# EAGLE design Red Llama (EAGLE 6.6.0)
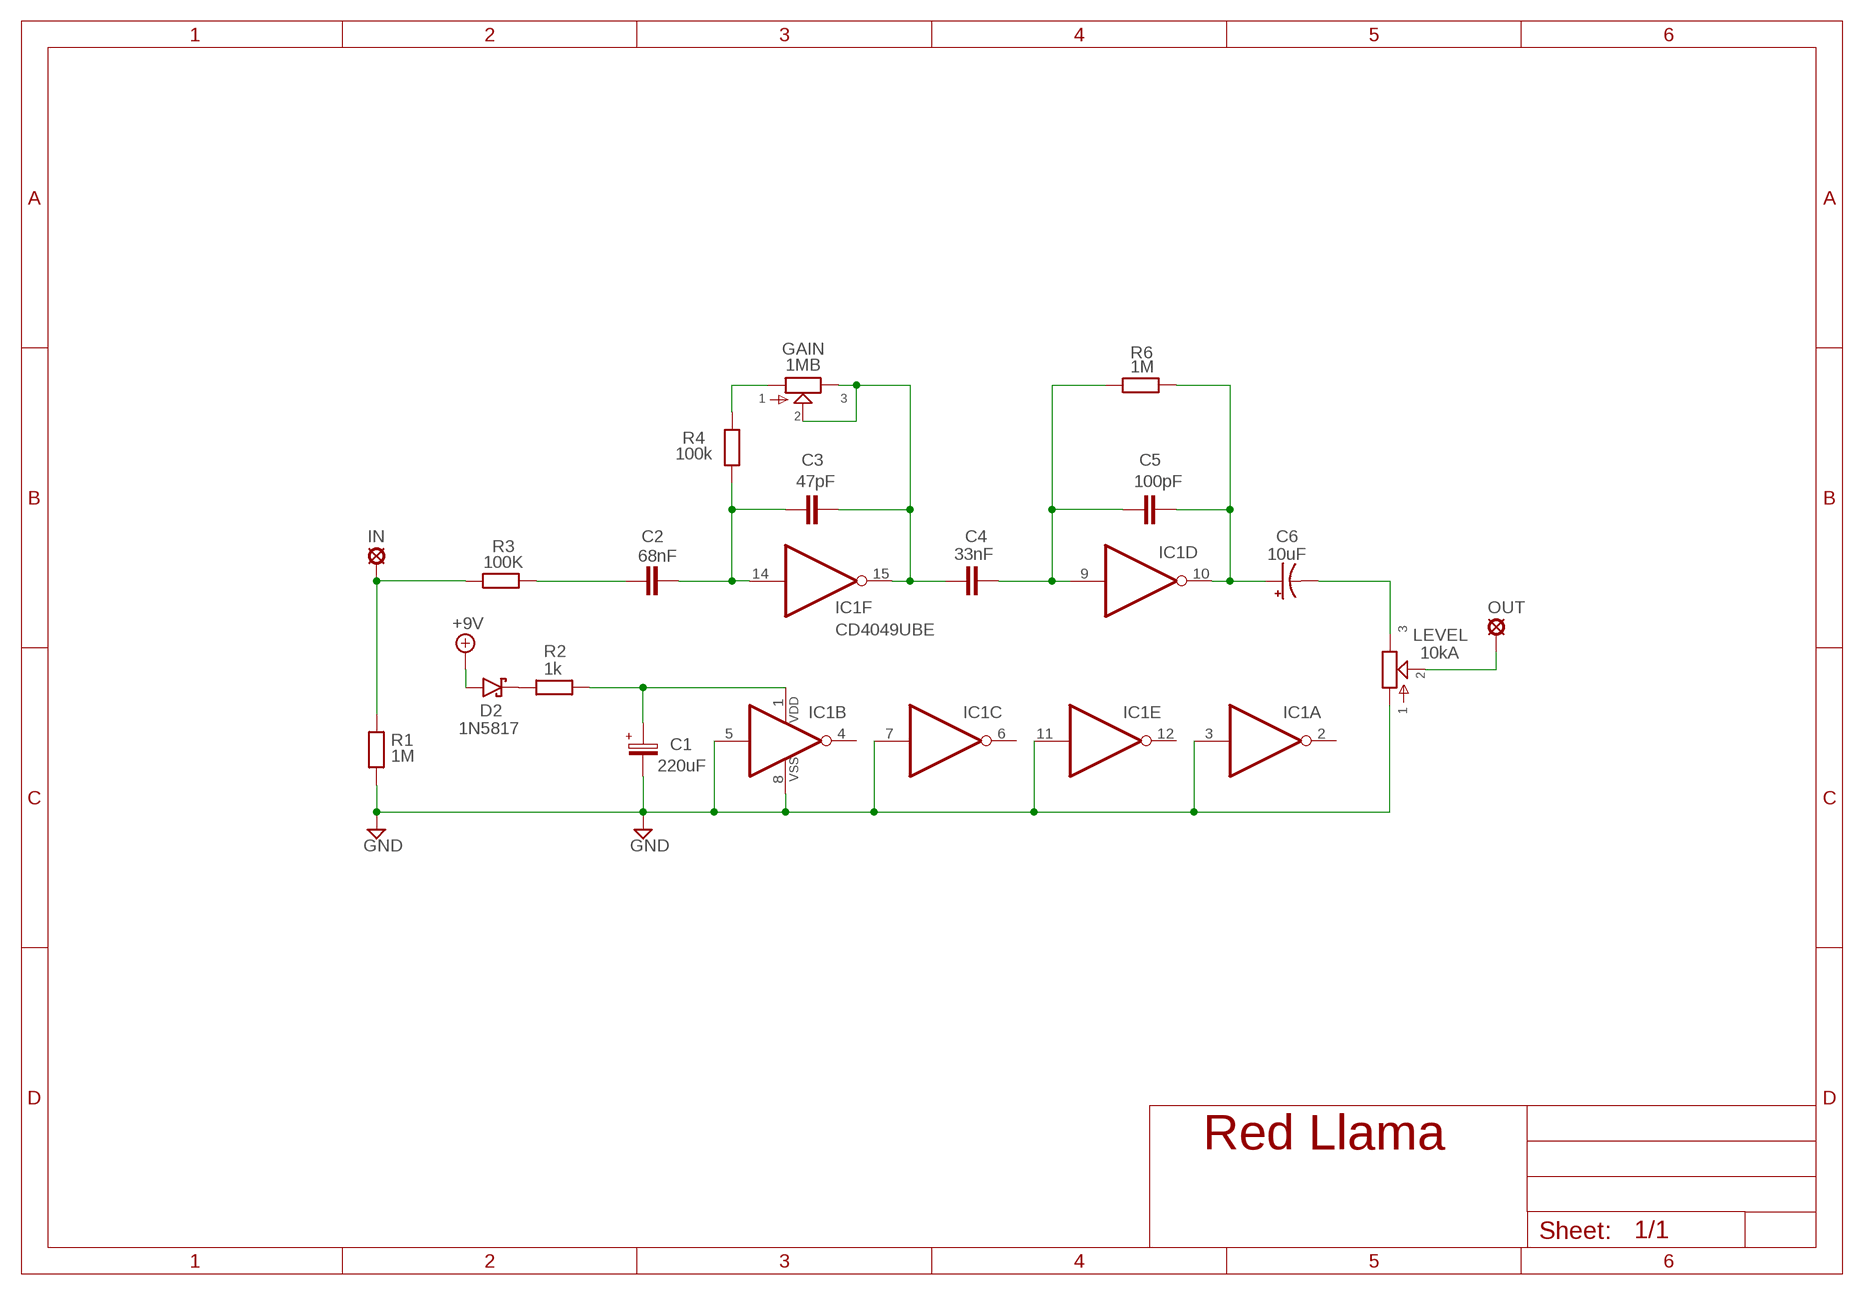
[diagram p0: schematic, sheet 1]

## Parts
+9V  +9V  +9V(T)1  [ROUND]
C1  220uF  063-EU  [063_025]
C2  68nF  10NF-47NF"  [4,5MM]
C3  47pF  050X030_0251  [050X030_025]
C4  33nF  10NF-47NF"  [4,5MM]
C5  100pF  050X030_0251  [050X030_025]
C6  10uF  044A2  [044A_2]
D2  1N5817  [DO41-3]
GAIN  1MB  POT-EU16MM  [16MM]
GND  GND  GND(T)1  [ROUND]
GND2  GND  GND(T)1  [ROUND]
IC1  CD4049UBE  [DIL16]
IN  MCS10B  [MCS10B]
LEVEL  10kA  POT-EU16MM  [16MM]
OUT  MCS10B  [MCS10B]
R1  1M  6MM-EU3  [R0207/3]
R2  1k  6MM-EU3  [R0207/3]
R3  100K  6MM-EU3  [R0207/3]
R4  100k  6MM-EU3  [R0207/3]
R6  1M  6MM-EU3  [R0207/3]

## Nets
+9V: +9V.1(+9V) D2.A
GND: C1.- GND2.1(GND) GND.1(GND) IC1.3(A:I) IC1.5(B:I) IC1.7(C:I) IC1.8(P:VSS) IC1.11(E:I) LEVEL.1 R1.1
N$1: LEVEL.2 OUT.MP
N$2: C4.2 C5.1 IC1.9(D:I) R6.1
N$3: IN.MP R1.2 R3.1
N$7: D2.C R2.1
N$8: GAIN.1 R4.2
N$9: C1.+ IC1.1(P:VDD) R2.2
N$18: C5.2 C6.1(+) IC1.10(D:O) R6.2
N$19: C3.2 C4.1 GAIN.2 GAIN.3 IC1.15(F:O)
N$20: C6.2(-) LEVEL.3
N$21: C2.2 C3.1 IC1.14(F:I) R4.1
N$24: C2.1 R3.2
Unconnected: IC1.2(A:O) IC1.4(B:O) IC1.6(C:O) IC1.12(E:O)

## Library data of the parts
+9V = gm-supply:+9V(T): +9V Voltage Supply
C1 = Elektrolyytit:063-EU
C2 C4 = Mylar Kondensaattorit:10NF-47NF: 10nF-47nF
C3 C5 = Keraamiset kondensaattorit:050X030_025: 47 - 120pF
C6 = gm-caps-tant:044A: .1 - 1.5µF
D2 = Diodit:1N5817
GAIN LEVEL = gm-pots:POT-EU
GND GND2 = gm-supply:GND(T): Ground
IC1 = Operaatiovahvistimet:CD4049UBE: Hex Inverting Buffer Used, for example, in the Red Llama, Three Legged Dog, and Hot Harmonics.
IN OUT = Padit:MCS10B: SOLDER PAD
R1-R4 R6 = Vastukset:6MM-EU: 6mm Resistors (European schematic symbol)

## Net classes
0 default: width 0.406 mm

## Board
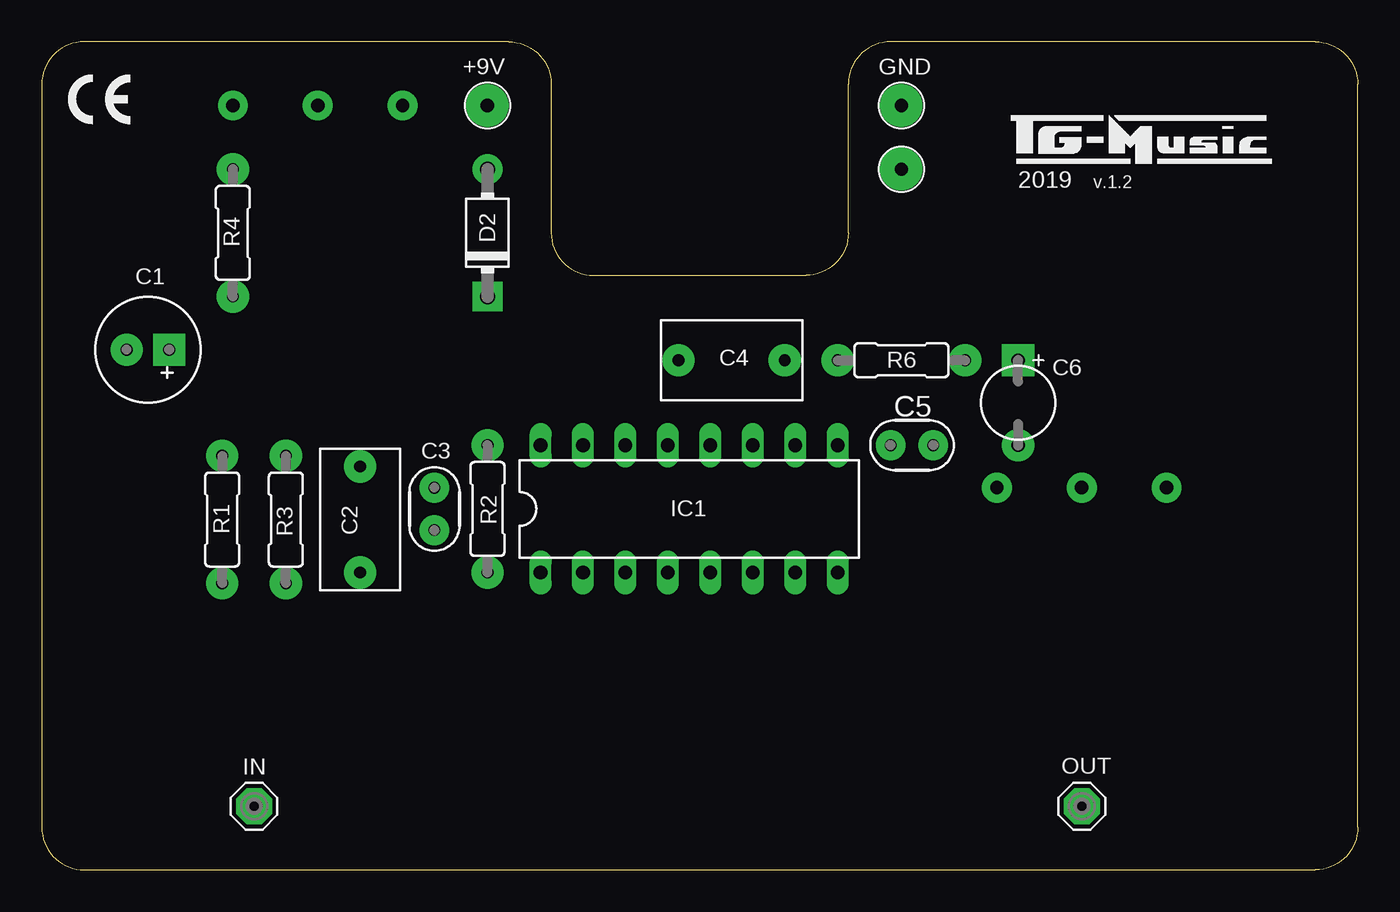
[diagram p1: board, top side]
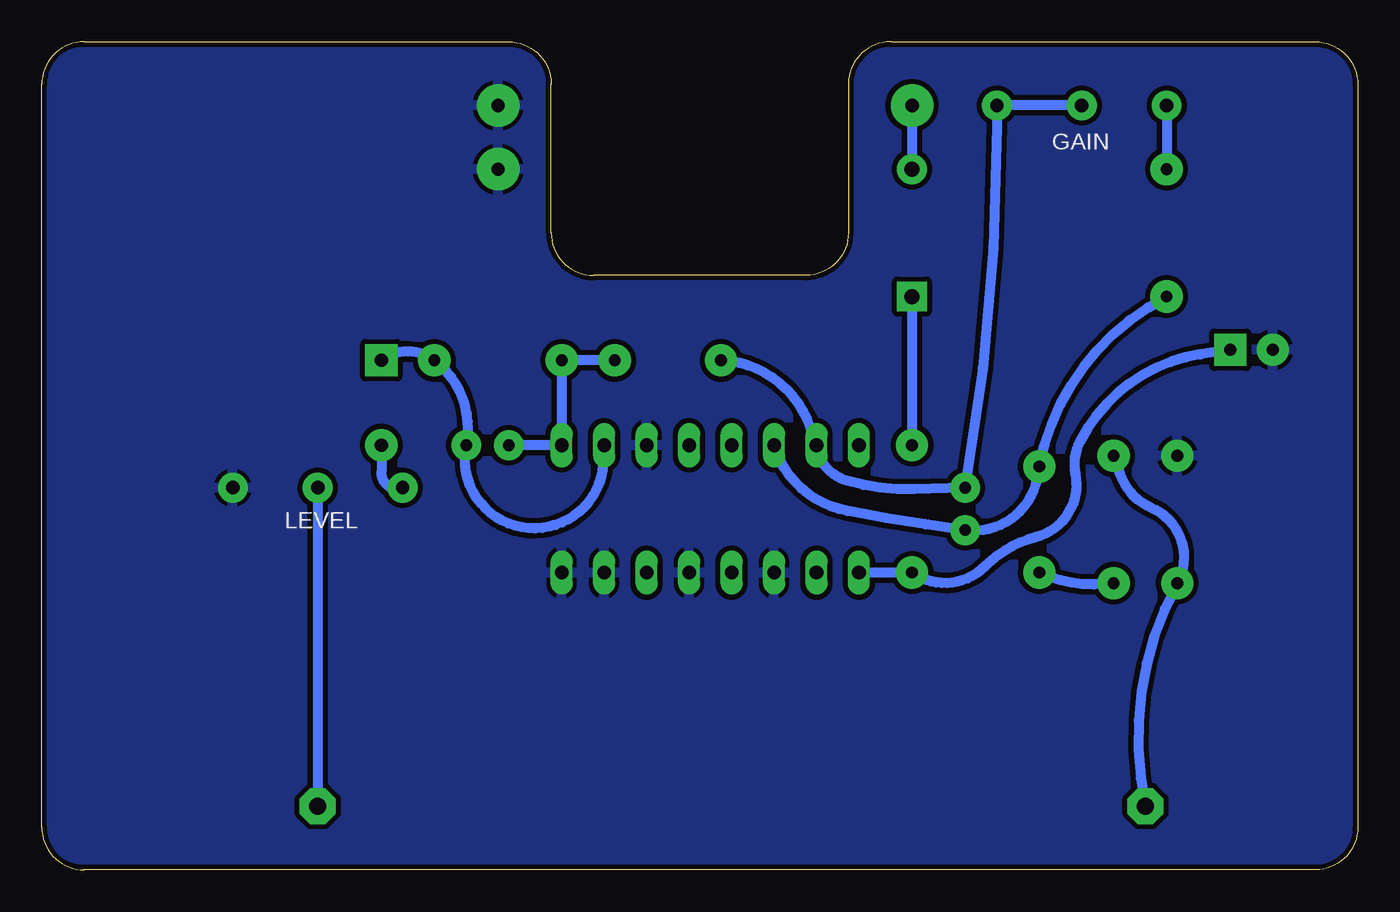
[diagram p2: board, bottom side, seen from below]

Size 78.74 x 49.53 mm. Coordinates in mm from the lower left corner, seen from the top.
Outline: 78.74,2.54 78.74,46.99 arc90 76.2,49.53 50.8,49.53 arc90 48.26,46.99 48.26,38.1 arc-90 45.72,35.56 33.02,35.56 arc-90 30.48,38.1 30.48,46.99 arc90 27.94,49.53 2.54,49.53 arc90 0,46.99 0,2.54 arc90 2.54,0 76.2,0 arc90 78.74,2.54
Copper layers (1*16): Top 0.035mm / dielectric 1.5mm / Bottom 0.035mm
Design rules "ITEADstudio": minimum track width 10mil, minimum drill 12mil, track to track 12mil, track to pad 12mil, pad to pad 12mil, via to via 12mil, smd to smd 0mil, copper to edge 12mil, drill to drill 12mil, minimum pad ring 10mil, minimum via ring 6mil, stop-mask expansion 4mil, vias tented up to drill 100mil, thermal gap 10mil

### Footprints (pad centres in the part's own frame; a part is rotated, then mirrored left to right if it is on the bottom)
ROUND = drill 0.8 pad 2.54: 1 0,0
063_025 = drill 0.7 pad 1.93 square: + -1.27,0 | drill 0.7 pad 1.93: - 1.27,0
4,5MM = drill 0.7 pad 1.93: 1 -3.175,0; 2 3.175,0
050X030_025 = drill 0.7 pad 1.778: 1 -1.27,0; 2 1.27,0
044A_2 = drill 0.8 pad 1.93 square: 1 -2.54,0 | drill 0.8 pad 1.93: 2 2.54,0
DO41-3 = drill 0.9 pad 1.778: A 3.81,0 | drill 0.9 pad 1.778 square: C -3.81,0
16MM = drill 0.8 pad 1.778: 1 5.08,0; 2 0,0; 3 -5.08,0
DIL16 = drill 0.813 long: 1 -8.89,-3.81; 2 -6.35,-3.81; 3 -3.81,-3.81; 4 -1.27,-3.81; 5 1.27,-3.81; 6 3.81,-3.81; 7 6.35,-3.81; 8 8.89,-3.81; 9 8.89,3.81; 10 6.35,3.81; 11 3.81,3.81; 12 1.27,3.81; 13 -1.27,3.81; 14 -3.81,3.81; 15 -6.35,3.81; 16 -8.89,3.81
MCS10B = drill 1.016 pad 2.159 octagon: MP 0,0
R0207/3 = drill 0.7 pad 1.93: 1 -3.81,0; 2 3.81,0

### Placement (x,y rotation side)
+9V  26.67,45.72 0 top
C1  6.35,31.11 180 top
C2  19.05,20.95 90 top
C3  23.5,21.59 90 top
C4  41.27,30.48 0 top
C5  52.07,25.4 0 top
C6  58.42,27.94 270 top
D2  26.67,38.1 90 top
GAIN  16.51,45.72 180 top
GND  51.44,45.72 0 top
GND2  51.44,41.91 0 top
IC1  38.73,21.59 0 top
IN  12.7,3.81 0 top
LEVEL  62.23,22.86 0 top
OUT  62.23,3.81 0 top
R1  10.79,20.95 270 top
R2  26.67,21.59 270 top
R3  14.61,20.95 270 top
R4  11.43,38.1 90 top
R6  51.44,30.48 0 top

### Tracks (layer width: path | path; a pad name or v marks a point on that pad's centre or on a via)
+9V
  Bottom 0.61: +9V.1 D2.A
GND
  pour Bottom: 0,2.54 0,46.99 arc-90 2.54,49.53 27.94,49.53 arc-90 30.48,46.99 30.48,38.1 arc90 33.02,35.56 45.72,35.56 arc90 48.26,38.1 48.26,46.99 arc-90 50.8,49.53 76.2,49.53 arc-90 78.74,46.99 78.74,1.91 arc-90 76.83,0 2.54,0 arc-90
N$1
  Bottom 0.61: LEVEL.2 OUT.MP
N$2
  Bottom 0.61: C5.1 IC1.9 R6.1 C4.2
N$3
  Bottom 0.61: R3.1 14.22,23.68 arc-47 12.34,21.66 arc95 R1.2 arc-41 IN.MP
N$7
  Bottom 0.61: D2.C R2.1
N$8
  Bottom 0.61: GAIN.1 R4.2
N$9
  Bottom 0.61: IC1.1 R2.2 arc-80 22.3,18.15 arc30 19.26,19.9 arc-86 16.9,23.68 arc39 16.62,25.65 arc54 9.41,30.84 C1.+
N$18
  Bottom 0.61: IC1.10 45.15,24.33 arc188 C5.2 arc-64 R6.2 arc-75 C6.1
N$19
  Bottom 0.61: C4.1 arc68 32.74,26.43 IC1.15 arc-67 30.57,23.28 arc-18 26.54,22.77 C3.2 arc-10 21.59,44.45 GAIN.3 GAIN.2
N$20
  Bottom 0.61: C6.2 58.42,23.81 arc-114 LEVEL.3
N$21
  Bottom 0.61: IC1.14 arc-62 30.55,21.47 arc-3 C3.1 arc-87 19.2,23.39 C2.2 arc51 R4.1
N$24
  Bottom 0.61: R3.2 15.11,17.1 arc30 C2.1

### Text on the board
tNames: 2019 | v.1.2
